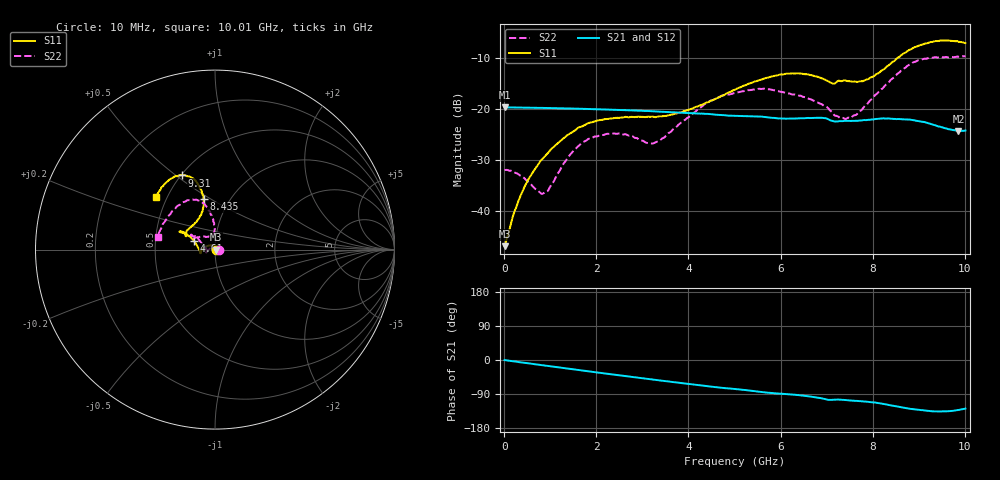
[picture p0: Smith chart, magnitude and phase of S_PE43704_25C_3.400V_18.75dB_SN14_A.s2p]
! Device ID: PE43704
! Dir: z:\PE43704\PE43704_Char_1_20130516\PE43704\AMB\3p400V\18p75dB
! Serial: 14
! Insertion: A
! Impedance: 50 ohm
! Temp: Amb
! VDD: 3.400V
! Attenuation Step: 18.75dB
! IDD: 1.139512e-01mA
#  Hz  S  RI  R  50
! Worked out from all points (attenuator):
!   401 points, 10 MHz to 10.01 GHz, reference 50 ohm
!   highest |S21| = -19.74 dB at 10 MHz (marker M1); lowest = -24.4 dB at 9.86 GHz (marker M2)
!   lowest |S11| = -46.9 dB at 10 MHz (marker M3), VSWR 1.01, Z = 50.5 + j0.0383 ohm
!   |S11| at or under -10 dB: start of sweep to 8.547 GHz
!   |S22| runs from -36.7 to -9.7 dB; largest |S21 - S12| = 0.0011
!   S11 on the Smith chart (normalised r, x): 10 MHz: 1.01, +0.00; 4.61 GHz: 0.79, +0.08; 8.435 GHz: 0.76, +0.46; 9.31 GHz: 0.51, +0.53; 10.01 GHz: 0.44, +0.32
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1e7  0.00448 0.00038  0.103 -0.000379  0.103 -0.000348  0.025 0.000182
2.35e8  0.00247 0.00984  0.1024 -0.00726  0.1024 -0.00719  0.0225 0.00714
4.1e8  -0.00167 0.0158  0.1015 -0.0126  0.1015 -0.0123  0.0181 0.0114
8.6e8  -0.0231 0.0239  0.0985 -0.025  0.0985 -0.025  -0.00278 0.0147
1.41e9  -0.0544 0.0148  0.0922 -0.0395  0.0923 -0.0395  -0.0344 0.00105
1.685e9  -0.0666 0.00562  0.0883 -0.0462  0.0884 -0.0462  -0.0451 -0.00956
2.36e9  -0.079 -0.0152  0.0766 -0.0604  0.0766 -0.0603  -0.0516 -0.0243
3.135e9  -0.0814 -0.018  0.0605 -0.0729  0.0604 -0.0729  -0.0454 -0.00736
3.36e9  -0.0833 -0.012  0.0553 -0.0754  0.0555 -0.0754  -0.0479 0.00274
4.61e9  -0.1169 0.0481  0.0271 -0.0827  0.0274 -0.0828  -0.1057 0.0703
5.01e9  -0.1368 0.0694  0.0196 -0.0829  0.0198 -0.0829  -0.1221 0.0737
5.685e9  -0.1753 0.0955  0.00594 -0.0824  0.00589 -0.0823  -0.1318 0.0824
6.685e9  -0.1896 0.0956  -0.0101 -0.0805  -0.0101 -0.0807  -0.1012 0.0678
7.135e9  -0.1571 0.0798  -0.0197 -0.0731  -0.0194 -0.0729  -0.0547 0.0714
7.485e9  -0.1431 0.1189  -0.0216 -0.0728  -0.0216 -0.0729  -0.0219 0.0785
7.86e9  -0.0964 0.1663  -0.0262 -0.0727  -0.0263 -0.0728  -0.00302 0.1081
8.36e9  -0.0625 0.2616  -0.0388 -0.0698  -0.0386 -0.07  -0.0159 0.1834
8.435e9  -0.0636 0.2811  -0.0404 -0.0684  -0.0406 -0.0687  -0.0243 0.1972
8.86e9  -0.1026 0.3757  -0.0492 -0.0597  -0.0486 -0.06  -0.08 0.2692
9.31e9  -0.1831 0.4135  -0.0497 -0.0488  -0.0495 -0.0487  -0.1707 0.2662
9.86e9  -0.3021 0.336  -0.0403 -0.0448  -0.0406 -0.0446  -0.2947 0.13
1.001e10  -0.3278 0.2916  -0.0378 -0.0479  -0.0386 -0.0477  -0.3188 0.0712
